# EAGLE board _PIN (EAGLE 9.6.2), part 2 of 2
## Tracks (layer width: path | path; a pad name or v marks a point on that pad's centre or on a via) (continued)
G11  (via drill 0.35) (continued)
  Top 0.152: D192.4 5.08,13.9 5.5,14.33 8.02,14.33 | 35.08,14.33 31.99,14.33 | 31.99,14.33 29.21,14.33 | 14.05,14.33 11.11,14.33 | 11.11,14.33 8.02,14.33 | D180.4 41.04,13.79 41.04,14.33 | D182.4 35.08,14.32 35.08,14.33 | D183.4 31.99,13.84 31.99,14.33 | D184.4 29.07,14.19 29.21,14.33 | D188.4 17.07,14.26 17.14,14.33 | D189.4 14.07,13.89 | 14.07,13.89 14.07,14.3 14.05,14.33 | D190.4 11.07,14.29 11.11,14.33 | D191.4 8.02,13.81 8.02,14.33 | 41.04,14.33 40.13,14.33 39.37,14.33 39.34,14.37 38.1,14.37 | 38.1,14.37 37.17,14.37 37.13,14.33 36.37,14.33 35.08,14.33 | 17.14,14.33 15.19,14.33 15.18,14.34 14.68,14.34 14.67,14.33 14.05,14.33 | v14.02,13.75 14.02,13.84 14.07,13.89 | D181.4 38.08,14.34 38.1,14.37 | 29.21,14.33 28.16,14.33 27.4,14.33 27.39,14.34 26.19,14.34 | 26.19,14.34 25.15,14.34 25.14,14.33 24.39,14.33 24.38,14.34 23.1,14.34 | 23.1,14.34 22.14,14.34 22.13,14.33 21.37,14.33 21.36,14.34 20.08,14.34 | 20.08,14.34 19.12,14.34 19.11,14.33 18.36,14.33 17.14,14.33 | D187.4 20.07,14.33 20.08,14.34 | D186.4 23.07,14.31 23.1,14.34 | D185.4 26.07,14.22 26.19,14.34 | D179.4 42.92,13.75 42.34,14.33 41.04,14.33
  Bottom 0.152: v14.02,13.75 13.49,13.22 13.49,9.51 13.54,9.46 13.54,8.96 13.49,8.9 13.49,6.55 13.53,6.52 13.53,5.78 P1.34
G12  (via drill 0.35)
  Top 0.152: D148.4 8.07,10.9 8.51,11.33 11.11,11.33 | 32.07,11.33 29.05,11.33 | 29.05,11.33 25.96,11.33 | 25.96,11.33 23.1,11.33 | 23.1,11.33 20,11.33 | 16.99,11.33 14.21,11.33 | 14.21,11.33 11.11,11.33 | D138.4 38.08,11.22 38.18,11.33 | D139.4 35.08,11.24 35.16,11.33 | D140.4 32.07,10.76 32.07,11.33 | D141.4 29.05,10.77 29.05,11.33 | D142.4 25.96,10.87 25.96,11.33 | D143.4 23.07,11.3 23.1,11.33 | D144.4 20,10.82 20,11.33 | D146.4 14.07,11.2 14.21,11.33 | D147.4 11.07,11.29 11.11,11.33 | 16.99,11.33 16.99,10.84 D145.4 v17.02,10.75 | D137.4 40.93,10.9 40.15,10.9 39.84,11.2 39.48,11.2 39.34,11.33 38.18,11.33 | 38.18,11.33 37.15,11.33 37.13,11.31 36.37,11.31 36.36,11.33 35.16,11.33 | 35.16,11.33 34.13,11.33 34.11,11.31 34.1,11.33 32.07,11.33 | 20,11.33 16.99,11.33
  Bottom 0.152: P1.37 17.5,8.45 17.02,8.93 v17.02,10.75
G13  (via drill 0.35)
  Top 0.152: D149.4 37.5,8.33 35.16,8.33 | D158.4 11.07,7.9 11.51,8.33 14.05,8.33 | 31.99,8.33 28.97,8.33 | 23.02,8.33 20,8.33 | 20,8.33 17.07,8.33 | 17.07,8.33 14.05,8.33 | D154.4 23.1,7.73 23.1,7.48 23.02,7.56 v23.02,7.78 23.02,8.33 | D155.4 20.07,8.26 20,8.33 | 17.07,8.08 D156.4 17.07,8.33 | D157.4 14.07,8.3 14.05,8.33 | D152.4 29.07,8.22 28.97,8.33 | D151.4 31.99,7.84 31.99,8.33 | D150.4 35.08,8.24 35.16,8.33 | D153.4 26.07,8.29 26.11,8.33 | 31.99,8.33 35.16,8.33 | 28.97,8.33 28.19,8.33 28.16,8.3 27.4,8.3 27.37,8.33 26.11,8.33 | 23.02,8.33 23.65,8.33 23.68,8.36 24.33,8.36 24.39,8.3 25.14,8.3 25.18,8.33 26.11,8.33
  Bottom 0.152: P1.40 v23.02,7.77 v23.02,7.78
G14  (via drill 0.35)
  Top 0.152: D164.4 17.37,5.05 17.37,5.2 17.5,5.33 18.34,5.33 18.36,5.32 20.08,5.32 | 23.18,5.33 20.5,5.33 20.5,5.32 20.08,5.32 | 23.18,5.33 26.04,5.33 | 26.04,5.33 28.97,5.33 | D160.4 28.97,4.85 | 28.97,4.85 28.97,5.33 | D161.4 26.07,5.29 26.04,5.33 | D162.4 23.07,5.23 23.18,5.33 | D163.4 20.07,5.31 20.08,5.32 | D159.4 31.5,5.33 28.97,5.33 | v29.02,4.75 28.97,4.8 28.97,4.85
  Bottom 0.152: P1.43 28.65,2.83 28.88,3.06 28.88,4.61 v29.02,4.75
GND  (via drill 0.35)
  Top 0.305: v22.32,47.89 22.25,47.82 C10.1 | U1.6 25.48,47.7 25.14,47.35 v24.84,47.05
  Bottom 0.305: P1.74 37.38,45.31 34.52,45.31 33.1,46.73 30.54,46.73 C9.1 29.13,48.15 27.35,48.15 26.75,47.55 26.75,46.39 26.34,45.97 24.84,45.97 | v22.32,47.89 23.14,47.06 23.14,46.4 23.57,45.97 24.84,45.97 | 24.84,45.97 24.84,45.98 v24.84,47.05
  other vias: 29.25,48.02
N$38
  Top 0.305: U1.3 U1.4
N$40  (via drill 0.35)
  Top 0.152: R11.1 18.81,47.33 v18.81,46.75 | U1.5 27.91,47.88 C9.2 27.86,47.83 v27.86,47.47
  Bottom 0.152: v18.81,46.75 19.46,46.1 19.46,45 19.85,44.61 20.48,44.61 20.68,44.81 20.68,45.45 21.31,46.07 22.19,46.07 22.67,45.59 26.78,45.59 27.86,46.67 v27.86,47.47
R0  (via drill 0.35)
  Top 0.152: D1.1 31.46,45.87 29.13,45.87 | D2.1 29.13,45.31 29.13,45.87 | D3.1 26.07,45.83 26.11,45.87 | D4.1 23.07,45.84 23.1,45.87 | 23.1,45.87 23.53,45.87 23.57,45.83 24.34,45.83 24.35,45.83 25.34,45.83 25.38,45.87 26.11,45.87 | D5.1 | D6.1 17.07,45.1 17.54,44.64 19.46,44.64 D5.1 | 26.11,45.87 27.26,45.87 27.28,45.85 28.9,45.85 28.91,45.87 29.13,45.87 | 23.1,45.87 20.56,45.87 20.52,45.83 20.5,45.83 20.07,45.39 D5.1
  Bottom 0.152: P1.3 20.07,47.53 D5.1
  other vias: 20.07,45.25
R1  (via drill 0.35)
  Top 0.152: D16.1 11.07,42.4 11.51,42.83 13.03,42.83 13.04,42.83 14.13,42.83 | 20.08,42.83 23.1,42.83 | 29.05,42.83 32.07,42.83 | D8.1 35.08,42.83 | D9.1 32.08,42.82 32.07,42.83 | D10.1 29.07,42.8 29.05,42.83 | D11.1 26.07,42.79 26.04,42.83 | D12.1 23.07,42.8 23.1,42.83 | D13.1 20.07,42.82 20.08,42.83 | D14.1 | D14.1 17.07,42.82 17.07,42.83 | D15.1 14.07,42.77 14.13,42.83 | 35.08,42.83 36.49,42.83 36.5,42.83 37.49,42.83 D7.1 | 32.07,42.83 33.48,42.83 33.99,42.83 35.08,42.83 | 26.04,42.83 27.52,42.83 27.53,42.83 28.03,42.83 28.04,42.83 29.05,42.83 | 23.1,42.83 24.51,42.83 25.02,42.83 26.04,42.83 | 17.07,42.83 18.48,42.83 18.98,42.83 18.99,42.83 20.08,42.83 | 14.13,42.83 15.54,42.83 16.05,42.83 17.07,42.83 | D14.1
  Bottom 0.152: P1.6 15.83,46.81 15.12,46.1 15.12,44.2 D14.1
  other vias: 17.07,42.25
R2  (via drill 0.35)
  Top 0.152: D28.1 8.07,39.4 8.57,39.9 10.01,39.9 10.08,39.83 11.19,39.83 | D17.1 40.5,39.83 38.02,39.83 | 11.19,39.83 14.13,39.83 | 14.13,39.83 17.07,39.83 | 17.07,39.83 20.08,39.83 | 20.08,39.83 23.02,39.83 | 23.02,39.83 26.04,39.83 | 26.04,39.83 29.05,39.83 | 29.05,39.83 31.99,39.83 | 31.99,39.83 35,39.83 | 35,39.83 38.02,39.83 | D18.1 38.02,39.3 38.02,39.83 | D19.1 35.08,39.76 35,39.83 | D20.1 32.08,39.74 31.99,39.83 | D21.1 29.07,39.8 29.05,39.83 | D22.1 26.07,39.79 26.04,39.83 | D23.1 23.07,39.77 23.02,39.83 | D24.1 20.07,39.82 20.08,39.83 | D25.1 17.07,39.82 17.07,39.83 | D26.1 14.07,39.77 14.13,39.83 | D27.1 | D27.1 11.07,39.71 11.19,39.83 | D27.1
  Bottom 0.152: P1.9 11.07,44.3 D27.1
  other vias: 11.07,39.25
R3  (via drill 0.35)
  Top 0.152: D42.1 5.08,36.4 5.5,36.83 6.44,36.83 6.5,36.88 7,36.88 7.05,36.83 8.1,36.83 | D29.1 43.5,36.83 41.04,36.83 | 8.1,36.83 11.11,36.83 | 14.13,36.83 16.99,36.83 | 16.99,36.83 20.08,36.83 | 20.08,36.83 23.02,36.83 | 23.02,36.83 26.19,36.83 | 26.19,36.83 29.13,36.83 | 29.13,36.83 32.07,36.83 | 32.07,36.83 35.16,36.83 | 35.16,36.83 38.02,36.83 | 38.02,36.83 41.04,36.83 | D30.1 41.04,36.29 41.04,36.83 | D31.1 38.02,36.3 38.02,36.83 | D32.1 35.08,36.74 35.16,36.83 | D33.1 32.07,36.26 32.07,36.83 | D34.1 29.07,36.77 29.13,36.83 | D35.1 26.07,36.71 26.19,36.83 | D36.1 23.07,36.77 23.02,36.83 | D38.1 17.07,36.74 16.99,36.83 | D39.1 14.07,36.77 14.13,36.83 | D40.1 11.07,36.79 11.11,36.83 | D41.1 | D41.1 8.07,36.81 8.1,36.83 | D37.1 20.07,36.82 20.08,36.83 | 11.11,36.83 12.47,36.83 12.53,36.88 13.03,36.88 13.08,36.83 14.13,36.83 | D41.1
  Bottom 0.152: D41.1 8.07,36.58 8.22,36.73 8.22,39.19 P1.12
  other vias: 8.07,36.25
R4  (via drill 0.35)
  Top 0.152: D165.1 43.5,33.83 41.04,33.83 | 8.02,33.83 5.5,33.83 5.08,33.4 D178.1 v5.07,33.26 | 17.14,33.83 20.16,33.83 | 22.94,33.83 26.11,33.83 | 26.11,33.83 29.13,33.83 | 35.08,33.83 38.1,33.83 | 38.1,33.83 41.04,33.83 | D166.1 41.04,33.29 41.04,33.83 | D167.1 38.08,33.8 38.1,33.83 | D168.1 35.08,33.82 35.08,33.83 | D169.1 32.08,33.82 32.07,33.83 | D170.1 29.07,33.77 29.13,33.83 | D171.1 26.07,33.79 26.11,33.83 | D172.1 23.07,33.69 22.94,33.83 | D173.1 20.07,33.74 20.16,33.83 | D174.1 17.07,33.76 17.14,33.83 | D175.1 14.07,33.72 13.97,33.83 | D176.1 11.07,33.71 11.19,33.83 | D177.1 8.07,33.77 8.02,33.83 | 32.07,33.83 33.45,33.83 33.48,33.87 33.99,33.87 34.02,33.83 35.08,33.83 | 29.13,33.83 30.43,33.83 30.47,33.87 30.97,33.87 31.01,33.83 32.07,33.83 | 20.16,33.83 21.46,33.83 21.5,33.87 22,33.87 22.04,33.83 22.94,33.83 | 13.97,33.83 15.51,33.83 15.54,33.87 16.05,33.87 16.08,33.83 17.14,33.83 | 11.19,33.83 12.49,33.83 12.53,33.87 13.03,33.87 13.07,33.83 13.97,33.83 | 8.02,33.83 9.47,33.83 9.51,33.87 10.01,33.87 10.05,33.83 11.19,33.83
  Bottom 0.152: P1.15 5.07,34.53 v5.07,33.26
R5  (via drill 0.35)
  Top 0.152: 2.08,30.4 2.52,30.85 2.54,30.85 2.55,30.84 3.99,30.84 4,30.83 5.24,30.83 | D58.1 2.08,30.4 | D43.1 46.5,30.83 44.13,30.83 | 8.18,30.83 11.11,30.83 | 11.11,30.83 14.05,30.83 | 14.05,30.83 16.99,30.83 | 38.18,30.83 41.04,30.83 | 41.04,30.83 44.13,30.83 | D52.1 20.07,30.82 20.08,30.83 | D53.1 17.07,30.74 16.99,30.83 | D54.1 14.07,30.8 14.05,30.83 | D55.1 11.07,30.79 11.11,30.83 | D48.1 32.08,30.76 32.15,30.83 | D47.1 35.08,30.82 35.08,30.83 | D49.1 29.07,30.77 29.13,30.83 | D50.1 26.07,30.79 26.11,30.83 | D51.1 23.07,30.8 23.1,30.83 | D46.1 38.08,30.72 38.18,30.83 | D45.1 41.04,30.29 41.04,30.83 | D44.1 44.08,30.77 44.13,30.83 | D57.1 5.08,30.66 5.24,30.83 | D56.1 8.07,30.73 8.18,30.83 | 35.08,30.83 36.48,30.83 36.5,30.85 37,30.85 37.02,30.83 38.18,30.83 | 32.15,30.83 33.46,30.83 33.48,30.85 33.99,30.85 34.01,30.83 35.08,30.83 | 26.11,30.83 27.51,30.83 27.53,30.85 28.03,30.85 28.05,30.83 29.13,30.83 | 29.13,30.83 30.45,30.83 30.47,30.85 30.97,30.85 30.99,30.83 32.15,30.83 | 23.1,30.83 24.49,30.83 24.51,30.85 25.02,30.85 25.04,30.83 26.11,30.83 | 20.08,30.83 21.48,30.83 21.5,30.85 22,30.85 22.02,30.83 23.1,30.83 | 16.99,30.83 18.46,30.83 18.48,30.85 18.98,30.85 19,30.83 20.08,30.83 | 5.24,30.83 6.47,30.83 6.5,30.85 7,30.85 7.02,30.83 8.18,30.83 | P1.18 1.79,30.69 2.08,30.4
  other vias: 1.67,30.69
R6  (via drill 0.35)
  Top 0.152: D74.1 2.08,27.4 2.51,27.83 3.98,27.83 3.99,27.83 | D59.1 46.5,27.83 44.05,27.83 | 5.08,27.83 8.1,27.83 | 11.03,27.83 14.13,27.83 | 17.14,27.83 20.16,27.83 | 20.16,27.83 23.1,27.83 | 38.1,27.83 41.04,27.83 | 41.04,27.83 44.05,27.83 | D73.1 5.08,27.82 5.08,27.83 | D71.1 11.07,27.79 11.03,27.83 | D72.1 8.07,27.81 8.1,27.83 | D69.1 17.07,27.76 17.14,27.83 | D70.1 14.07,27.77 14.13,27.83 | D68.1 20.07,27.74 20.16,27.83 | D67.1 23.07,27.8 23.1,27.83 | D66.1 26.07,27.79 26.11,27.83 | D65.1 29.07,27.73 28.97,27.83 | D64.1 32.08,27.76 32.15,27.83 | D63.1 35.08,27.74 35.16,27.83 | D62.1 38.08,27.8 38.1,27.83 | D61.1 41.08,27.79 41.04,27.83 | D60.1 44.08,27.81 44.05,27.83 | 35.16,27.83 36.49,27.83 36.5,27.83 37,27.83 37.01,27.83 38.1,27.83 | 32.15,27.83 33.48,27.83 33.99,27.83 35.16,27.83 | 26.11,27.83 27.53,27.83 28.03,27.83 28.04,27.83 28.97,27.83 | 28.97,27.83 30.46,27.83 30.47,27.83 30.97,27.83 32.15,27.83 | 23.1,27.83 24.51,27.83 25.02,27.83 26.11,27.83 | 14.13,27.83 15.54,27.83 16.05,27.83 17.14,27.83 | 8.1,27.83 9.51,27.83 10.01,27.83 10.02,27.83 11.03,27.83 | 3.99,27.83 5.08,27.83 | v3.97,27.3 3.99,27.32 3.99,27.83
  Bottom 0.152: P1.21 3.21,27.3 v3.97,27.3
R7  (via drill 0.35)
  Top 0.152: D75.1 46.5,24.83 44.05,24.83 | D90.1 2.08,24.4 2.5,24.83 4.05,24.83 | 44.05,24.83 41.04,24.83 | 41.04,24.83 38.1,24.83 | 35.08,24.83 31.99,24.83 | 31.99,24.83 29.13,24.83 | 29.13,24.83 26.11,24.83 | 26.11,24.83 23.18,24.83 | 23.18,24.83 20.08,24.83 | 20.08,24.83 17.07,24.83 | 11.11,24.83 8.1,24.83 | 8.1,24.83 5.08,24.83 | 5.08,24.83 4.05,24.83 | D88.1 8.07,24.81 8.1,24.83 | D89.1 5.08,24.82 5.08,24.83 | D83.1 23.07,24.73 23.18,24.83 | D84.1 20.07,24.82 20.08,24.83 | D85.1 17.07,24.82 17.07,24.83 | D86.1 14.07,24.77 14.13,24.83 | D87.1 11.07,24.79 11.11,24.83 | D81.1 29.07,24.77 29.13,24.83 | D80.1 32.08,24.74 31.99,24.83 | D79.1 35.08,24.82 35.08,24.83 | D78.1 38.08,24.8 38.1,24.83 | D77.1 41.08,24.79 41.04,24.83 | D76.1 44.08,24.81 44.05,24.83 | D82.1 26.07,24.79 26.11,24.83 | 38.1,24.83 36.21,24.83 36.18,24.86 35.68,24.86 35.65,24.83 35.08,24.83 | 17.07,24.83 16.11,24.83 16.05,24.9 15.54,24.9 15.48,24.83 14.13,24.83 | 14.13,24.83 13.1,24.83 13.03,24.9 12.53,24.9 12.46,24.83 11.11,24.83 | v4.05,24.21 4.05,24.83
  Bottom 0.152: P1.24 2.86,20.71 2.86,23.02 v4.05,24.21
R8  (via drill 0.35)
  Top 0.152: D106.1 2.08,21.4 2.5,21.83 5.16,21.83 | 5.16,21.83 8.1,21.83 | 8.1,21.83 11.03,21.83 | 11.03,21.83 14.13,21.83 | 14.13,21.83 17.07,21.83 | 17.07,21.83 20.24,21.83 | 20.24,21.83 23.1,21.83 | 23.1,21.83 26.04,21.83 | 26.04,21.83 28.97,21.83 | 28.97,21.83 31.99,21.83 | 38.02,21.83 41.12,21.83 | D92.1 44.05,21.27 44.05,21.83 | D93.1 41.08,21.79 41.12,21.83 | D94.1 38.08,21.77 38.02,21.83 | D95.1 35.08,21.82 35.08,21.83 | D96.1 32.08,21.74 31.99,21.83 | D105.1 | D105.1 5.08,21.74 5.16,21.83 | D104.1 8.07,21.81 8.1,21.83 | D103.1 11.03,21.29 11.03,21.83 | D102.1 14.07,21.77 14.13,21.83 | D101.1 17.07,21.82 17.07,21.83 | D100.1 20.07,21.66 20.24,21.83 | D99.1 23.07,21.8 23.1,21.83 | D98.1 26.07,21.79 26.04,21.83 | D97.1 29.07,21.73 28.97,21.83 | 41.12,21.83 41.65,21.83 41.68,21.86 42.18,21.86 42.21,21.83 44.05,21.83 | D91.1 47.06,21.26 47.06,21.76 46.47,22.36 45.96,22.36 45.43,21.83 44.05,21.83 | 35.08,21.83 36.45,21.83 36.5,21.88 37,21.88 37.05,21.83 38.02,21.83 | 35.08,21.83 34.44,21.83 34.39,21.88 33.89,21.88 33.84,21.83 31.99,21.83 | v5.07,21.25 D105.1
  Bottom 0.152: P1.27 4.42,15.04 4.42,20.6 v5.07,21.25
R9  (via drill 0.35)
  Top 0.152: 2.08,18.4 2.08,18.34 | 2.08,18.34 D122.1 | 43.97,18.83 41.04,18.83 | 20,18.83 16.99,18.83 | 14.13,18.83 10.95,18.83 | 10.95,18.83 8.18,18.83 | D120.1 | D120.1 8.07,18.73 8.18,18.83 | D119.1 11.07,18.71 10.95,18.83 | D118.1 14.07,18.77 14.13,18.83 | D117.1 16.99,18.34 16.99,18.83 | D116.1 20.07,18.76 20,18.83 | D115.1 23.02,18.31 23.02,18.83 | D114.1 26.07,18.79 26.11,18.83 | D113.1 29.07,18.77 29.13,18.83 | D112.1 32.07,18.26 32.07,18.83 | D111.1 35.08,18.66 35.24,18.83 | D110.1 38.08,18.8 38.1,18.83 | D109.1 41.04,18.29 41.04,18.83 | D108.1 43.97,18.35 43.97,18.83 | 43.97,18.83 44.65,18.83 44.68,18.86 46.47,18.86 D107.1 | 41.04,18.83 40.12,18.83 40,18.94 39.5,18.94 39.39,18.83 38.1,18.83 | 38.1,18.83 37.03,18.83 37,18.86 36.5,18.86 36.47,18.83 35.24,18.83 | 35.24,18.83 34.02,18.83 33.99,18.86 33.48,18.86 33.45,18.83 32.07,18.83 | 29.13,18.83 28.07,18.83 28.03,18.86 27.53,18.86 27.5,18.83 26.11,18.83 | 32.07,18.83 31,18.83 30.97,18.86 30.47,18.86 30.43,18.83 30.21,18.83 30.18,18.86 29.68,18.86 29.65,18.83 29.13,18.83 | D120.1 | 26.11,18.83 25.05,18.83 25.02,18.86 24.51,18.86 24.48,18.83 23.02,18.83 | 23.02,18.83 22.11,18.83 22,18.94 21.5,18.94 21.38,18.83 20,18.83 | 16.99,18.83 16.08,18.83 16.05,18.86 15.54,18.86 15.51,18.83 14.13,18.83 | 8.18,18.83 7.03,18.83 7,18.86 6.5,18.86 6.46,18.83 5.16,18.83 | 2.08,18.34 2.37,18.63 2.37,18.7 2.5,18.83 5.16,18.83 | D121.1 5.08,18.74 5.16,18.83
  Bottom 0.152: D120.1 7.42,17.6 7.42,10.24 P1.30
  other vias: 8.07,18.25
R10  (via drill 0.35)
  Top 0.152: D136.1 5.08,15.4 5.55,15.88 6.37,15.88 6.38,15.87 8.1,15.87 | D123.1 43.46,15.87 41.12,15.87 | 8.1,15.87 11.03,15.87 | 11.03,15.87 14.05,15.87 | 14.05,15.87 17.14,15.87 | 17.14,15.87 20.16,15.87 | 20.16,15.87 23.18,15.87 | 23.18,15.87 26.04,15.87 | 26.04,15.87 29.13,15.87 | 29.13,15.87 32.07,15.87 | 32.07,15.87 35.08,15.87 | 35.08,15.87 38.1,15.87 | 38.1,15.87 41.12,15.87 | D125.1 38.08,15.84 38.1,15.87 | D124.1 41.08,15.82 41.12,15.87 | D126.1 35.08,15.86 35.08,15.87 | D128.1 29.07,15.81 29.13,15.87 | D129.1 26.07,15.83 26.04,15.87 | D130.1 23.07,15.76 23.18,15.87 | D131.1 20.07,15.78 20.16,15.87 | D132.1 17.07,15.8 17.14,15.87 | D133.1 14.07,15.84 14.05,15.87 | D134.1 | D134.1 11.07,15.82 11.03,15.87 | D135.1 8.07,15.85 8.1,15.87 | D127.1 32.07,15.26 32.07,15.87 | D134.1
  Bottom 0.152: P1.33 10.83,15.01 D134.1
  other vias: 11.07,15.25
R11  (via drill 0.35)
  Top 0.152: D192.1 5.08,12.4 5.51,12.83 7,12.83 8.18,12.83 | 8.18,12.83 11.11,12.83 | 11.11,12.83 14.05,12.83 | 20,12.83 23.1,12.83 | 38.1,12.83 41.04,12.83 | D181.1 38.08,12.8 38.1,12.83 | D180.1 41.08,12.79 41.04,12.83 | D182.1 35.08,12.76 35,12.83 | D183.1 32.07,12.26 32.07,12.83 | D184.1 29.07,12.69 29.21,12.83 | D185.1 25.96,12.37 25.96,12.83 | D186.1 23.07,12.8 23.1,12.83 | D187.1 20,12.32 20,12.83 | D188.1 | D188.1 17.07,12.68 17.22,12.83 | D189.1 14.05,12.28 14.05,12.83 | D190.1 11.07,12.79 11.11,12.83 | D191.1 8.07,12.73 8.18,12.83 | 35,12.83 36.5,12.83 37,12.83 38.1,12.83 | 41.04,12.83 41.65,12.83 41.68,12.86 43.47,12.86 D179.1 | 32.07,12.83 33.4,12.83 33.48,12.91 33.99,12.91 34.07,12.83 35,12.83 | 25.96,12.83 27.5,12.83 27.53,12.86 28.03,12.86 28.06,12.83 29.21,12.83 | 29.21,12.83 30.39,12.83 30.47,12.91 30.97,12.91 31.05,12.83 32.07,12.83 | D188.1 | 23.1,12.83 24.51,12.83 25.02,12.83 25.96,12.83 | 17.22,12.83 18.48,12.83 18.98,12.83 18.99,12.83 20,12.83 | 14.05,12.83 15.54,12.83 16.05,12.83 17.22,12.83
  Bottom 0.152: P1.36 16.51,3.71 16.51,10.4 16.41,10.5 16.41,11.6 D188.1
  other vias: 17.07,12.25
R12  (via drill 0.35)
  Top 0.152: D148.1 8.07,9.4 8.57,9.89 10.09,9.89 10.16,9.83 11.03,9.83 | D137.1 40.5,9.83 38.1,9.83 | 17.14,9.83 20.16,9.83 | 20.16,9.83 22.94,9.83 | 22.94,9.83 26.04,9.83 | 26.04,9.83 29.05,9.83 | D142.1 26.07,9.79 26.04,9.83 | D143.1 23.07,9.69 22.94,9.83 | D141.1 29.07,9.8 29.05,9.83 | D144.1 | D144.1 20.07,9.74 20.16,9.83 | D145.1 17.07,9.76 17.14,9.83 | D146.1 14.07,9.8 14.05,9.83 | D138.1 38.08,9.8 38.1,9.83 | D139.1 35.08,9.68 34.92,9.83 | D140.1 32.08,9.76 32.15,9.83 | 34.92,9.83 34.05,9.83 33.99,9.89 33.48,9.89 33.42,9.83 33.21,9.83 33.18,9.86 32.68,9.86 32.65,9.83 32.15,9.83 | 29.05,9.83 30.4,9.83 30.47,9.89 30.97,9.89 31.04,9.83 32.15,9.83 | 34.92,9.83 35.65,9.83 35.68,9.86 36.18,9.86 36.21,9.83 38.1,9.83 | D144.1 | 14.05,9.83 15.48,9.83 15.54,9.89 16.05,9.89 16.11,9.83 17.14,9.83 | D147.1 11.07,9.79 11.03,9.83 | 11.03,9.83 11.71,9.83 11.73,9.86 12.24,9.86 12.27,9.83 14.05,9.83
  Bottom 0.152: P1.39 21.16,1.91 20.07,2.99 D144.1
  other vias: 20.07,9.25
R13  (via drill 0.35)
  Top 0.152: D149.1 37.46,6.87 37.01,6.87 37,6.88 36.5,6.88 36.49,6.87 35.08,6.87 | D158.1 11.07,6.4 11.62,6.94 12.26,6.94 12.34,6.87 12.66,6.87 12.67,6.88 13.17,6.88 13.18,6.87 14.05,6.87 | 17.07,6.87 14.05,6.87 | D157.1 14.05,6.28 14.05,6.87 | D150.1 35.08,6.86 35.08,6.87 | D151.1 32.08,6.79 32.15,6.87 | D152.1 29.07,6.87 | D153.1 26.07,6.43 | 26.07,6.43 26.07,6.75 26.19,6.87 | D154.1 23.07,6.84 23.1,6.87 | D156.1 17.07,6.86 17.07,6.87 | D155.1 20.07,6.79 20,6.87 | 35.08,6.87 34,6.87 33.99,6.88 33.48,6.88 33.47,6.87 32.15,6.87 | 29.07,6.87 28.04,6.87 28.03,6.88 27.53,6.88 27.52,6.87 26.19,6.87 | v26.07,6.27 26.07,6.42 26.07,6.43 | 26.19,6.87 25.03,6.87 25.02,6.88 24.51,6.88 24.5,6.87 23.1,6.87 | 20,6.87 19,6.87 18.98,6.88 18.48,6.88 18.47,6.87 17.07,6.87 | 23.1,6.87 22.01,6.87 22,6.88 21.5,6.88 21.49,6.87 20,6.87 | 29.07,6.87 32.15,6.87
  Bottom 0.152: P1.42 26.07,1.88 v26.07,6.27
R14  (via drill 0.35)
  Top 0.152: D164.1 17.37,3.55 17.37,3.69 17.5,3.83 20.16,3.83 | 31.91,3.42 31.5,3.83 28.97,3.83 | 31.91,3.42 D159.1 | D160.1 28.97,3.35 28.97,3.83 | D161.1 26.07,3.79 26.11,3.83 | D162.1 23.07,3.77 23.02,3.83 | D163.1 20.07,3.74 20.16,3.83 | 26.11,3.83 27.5,3.83 27.53,3.86 28.03,3.86 28.07,3.83 28.97,3.83 | v32.07,3.25 31.91,3.41 31.91,3.42 | 23.02,3.83 24.48,3.83 24.51,3.86 25.02,3.86 25.05,3.83 26.11,3.83 | 20.16,3.83 21.46,3.83 21.5,3.86 22,3.86 22.03,3.83 23.02,3.83
  Bottom 0.152: P1.45 32.07,2.49 v32.07,3.25
SCL  (via drill 0.35)
  Top 0.152: U1.7 24.9,48.26 24.9,48.27 25.07,48.44 27.32,48.44 27.5,48.63 30.06,48.63 30.81,47.88 33.29,47.88 36.07,45.1 38.24,45.1 38.7,44.64 39.1,44.64 39.69,44.05 39.69,43.18 40.92,41.95 P1.71
  other vias: 41.92,41.95
SDA  (via drill 0.35)
  Top 0.152: U1.1 23.93,48.9 23.93,48.88 24.06,48.75 27.07,48.75 27.14,48.82 27.27,48.82 27.38,48.93 30.18,48.93 30.94,48.18 33.42,48.18 36.2,45.4 38.37,45.4 38.83,44.94 39.28,44.94 40.54,43.68 P1.72
  other vias: 40.54,43.23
